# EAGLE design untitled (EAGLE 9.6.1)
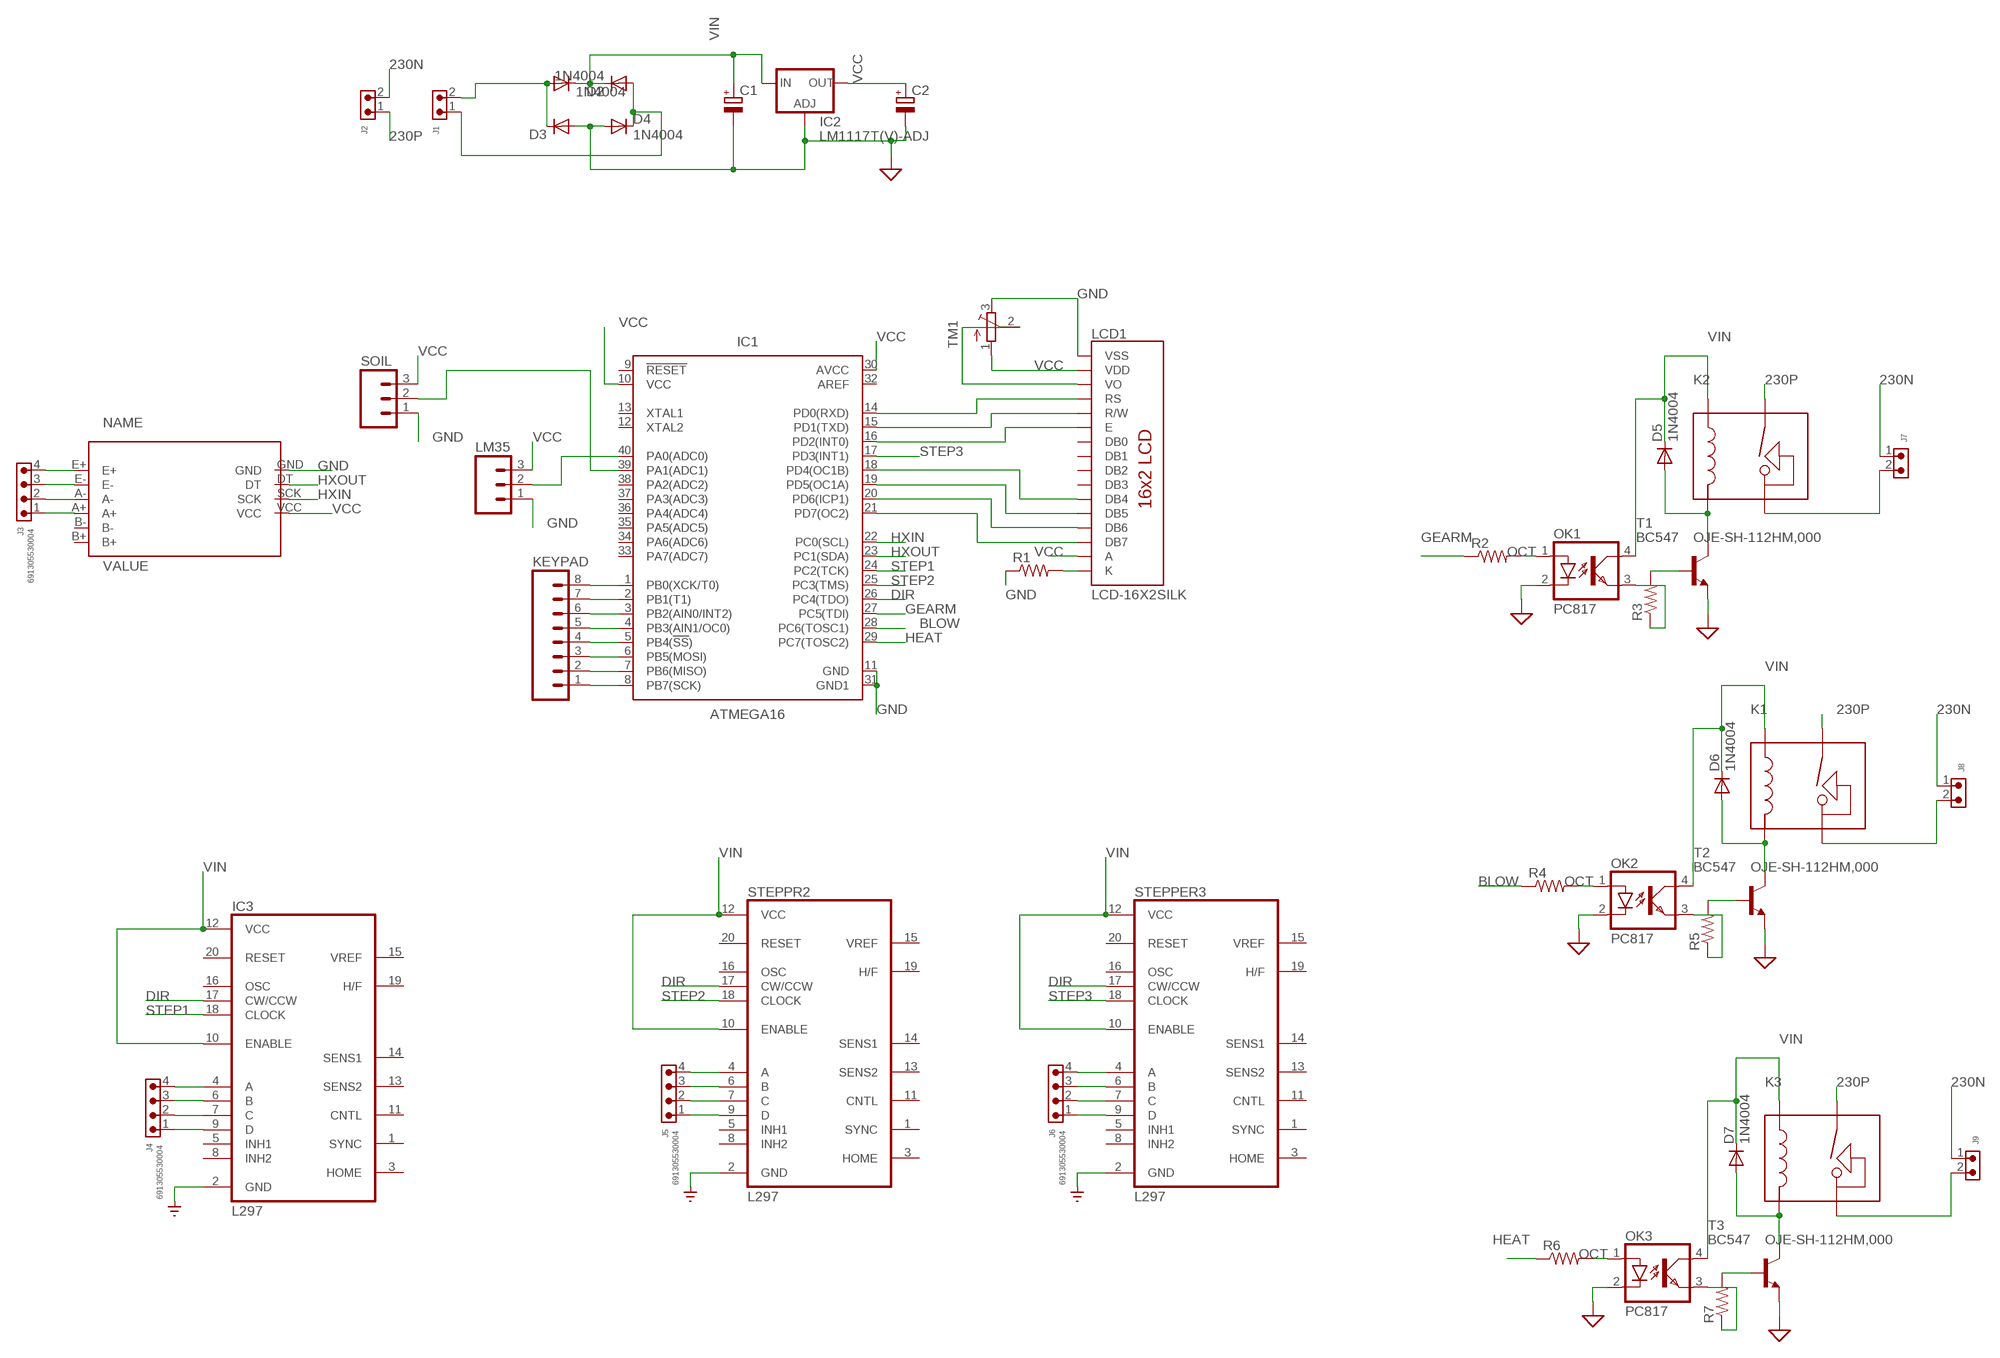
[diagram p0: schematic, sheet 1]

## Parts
C1  CPOL-EUE5-10.5  [E5-10,5]
C2  CPOL-EUE5-10.5  [E5-10,5]
D1  1N4004  [DO41-10]
D2  1N4004  [DO41-10]
D3  1N4004  [DO41-10]
D4  1N4004  [DO41-10]
D5  1N4004  [DO41-10]
D6  1N4004  [DO41-10]
D7  1N4004  [DO41-10]
IC1  ATMEGA16  ATMEGA32-16PU_DIP  [DIP1587W56P254L5229H482Q40B]
IC2  LM1117T(V)-ADJ  [TO220V]
IC3  L297  [DIL20]
J1  691305530002  [691305530002]
J2  691305530002  [691305530002]
J3  691305530004  691305530004  [691305530004]
J4  691305530004  691305530004  [691305530004]
J5  691305530004  691305530004  [691305530004]
J6  691305530004  691305530004  [691305530004]
J7  691305530002  [691305530002]
J8  691305530002  [691305530002]
J9  691305530002  [691305530002]
K1  OJE-SH-112HM,000  [OJE-SH-112HM,000]
K2  OJE-SH-112HM,000  [OJE-SH-112HM,000]
K3  OJE-SH-112HM,000  [OJE-SH-112HM,000]
KEYPAD  M08  [08P]
LCD1  LCD-16X2SILK  [LCD-16X2]
LM35  M03  [03P]
OK1  PC817  [DIL04]
OK2  PC817  [DIL04]
OK3  PC817  [DIL04]
R1  R-US_0207/9  [0207/9]
R2  R-US_0207/10  [0207/10]
R3  R-US_0207/10  [0207/10]
R4  R-US_0207/10  [0207/10]
R5  R-US_0207/10  [0207/10]
R6  R-US_0207/10  [0207/10]
R7  R-US_0207/10  [0207/10]
SOIL  M03  [03P]
STEPPER3  L297  [DIL20]
STEPPR2  L297  [DIL20]
T1  BC547  [TO92]
T2  BC547  [TO92]
T3  BC547  [TO92]
TM1  TRIMPOTTC33X  [TC33X]
U$3  HX711A  [HX711]

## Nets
230N: J2.2 J7.1 J8.1 J9.1
230P: J2.1 K1.NC K2.NC K3.NC
BLOW: IC1.28(PC6(TOSC1)) R4.1
DIR: IC1.26(PC4(TDO)) IC3.17(CW/CCW) STEPPER3.17(CW/CCW) STEPPR2.17(CW/CCW)
GEARM: IC1.27(PC5(TDI)) R2.1
GND: C1.- C2.- D3.A D4.A IC1.11(GND) IC1.31(GND1) IC2.1(ADJ) IC3.2(GND) LCD1.1(VSS) LM35.1 OK1.2(C) OK2.2(C) OK3.2(C) R1.1 SOIL.1 STEPPER3.2(GND) STEPPR2.2(GND) T1.1(E) T2.1(E) T3.1(E) TM1.3(E) U$3.GND ; supply symbol labelled SUP, SUPPLY0_GND_
HEAT: IC1.29(PC7(TOSC2)) R6.1
HXIN: IC1.22(PC0(SCL)) U$3.SCK
HXOUT: IC1.23(PC1(SDA)) U$3.DT
N$1: D1.A D3.C J1.2
N$2: D2.A D4.C J1.1
N$3: J3.4 U$3.E+
N$4: IC1.8(PB7(SCK)) KEYPAD.1
N$5: IC1.7(PB6(MISO)) KEYPAD.2
N$6: IC1.6(PB5(MOSI)) KEYPAD.3
N$7: IC1.5(PB4(!SS!)) KEYPAD.4
N$8: IC1.4(PB3(AIN1/OC0)) KEYPAD.5
N$9: J3.3 U$3.E-
N$10: J3.2 U$3.A-
N$11: J3.1 U$3.A+
N$12: IC1.3(PB2(AIN0/INT2)) KEYPAD.6
N$13: IC1.2(PB1(T1)) KEYPAD.7
N$14: IC1.1(PB0(XCK/T0)) KEYPAD.8
N$15: IC1.21(PD7(OC2)) LCD1.14(DB7)
N$16: IC1.20(PD6(ICP1)) LCD1.13(DB6)
N$17: IC1.19(PD5(OC1A)) LCD1.12(DB5)
N$18: IC1.18(PD4(OC1B)) LCD1.11(DB4)
N$19: IC1.14(PD0(RXD)) LCD1.4(RS)
N$20: IC1.15(PD1(TXD)) LCD1.5(R/W)
N$21: IC1.16(PD2(INT0)) LCD1.6(E)
N$22: IC3.4(A) J4.4
N$23: LCD1.3(VO) TM1.2(S)
N$24: IC3.6(B) J4.3
N$25: LCD1.16(K) R1.2
N$26: IC3.7(C) J4.2
N$27: IC3.9(D) J4.1
N$28: J5.4 STEPPR2.4(A)
N$29: J5.3 STEPPR2.6(B)
N$30: J5.2 STEPPR2.7(C)
N$31: J5.1 STEPPR2.9(D)
N$32: J6.4 STEPPER3.4(A)
N$33: J6.3 STEPPER3.6(B)
N$34: J6.2 STEPPER3.7(C)
N$35: J6.1 STEPPER3.9(D)
N$36: D5.A K2.A2 T1.3(C)
N$37: OK1.3(EMIT) R3.1
N$38: R3.2 T1.2(B)
N$39: IC1.40(PA0(ADC0)) LM35.2
N$40: J7.2 K2.NO
N$41: D6.A K1.A2 T2.3(C)
N$42: OK2.3(EMIT) R5.1
N$43: R5.2 T2.2(B)
N$44: IC1.39(PA1(ADC1)) SOIL.2
N$45: J8.2 K1.NO
N$46: D7.A K3.A2 T3.3(C)
N$47: OK3.3(EMIT) R7.1
N$48: R7.2 T3.2(B)
N$50: J9.2 K3.NO
OCT: OK1.1(A) OK2.1(A) OK3.1(A) R2.2 R4.2 R6.2
STEP1: IC1.24(PC2(TCK)) IC3.18(CLOCK)
STEP2: IC1.25(PC3(TMS)) STEPPR2.18(CLOCK)
STEP3: IC1.17(PD3(INT1)) STEPPER3.18(CLOCK)
VCC: C2.+ IC1.10(VCC) IC1.30(AVCC) IC2.2(OUT) LCD1.2(VDD) LCD1.15(A) LM35.3 SOIL.3 TM1.1(A) U$3.VCC
VIN: C1.+ D1.C D2.C D5.C D6.C D7.C IC2.3(IN) IC3.10(ENABLE) IC3.12(VCC) K1.A1 K2.A1 K3.A1 OK1.4(COL) OK2.4(COL) OK3.4(COL) STEPPER3.10(ENABLE) STEPPER3.12(VCC) STEPPR2.10(ENABLE) STEPPR2.12(VCC)
Unconnected: IC1.9(!RESET!) IC1.12(XTAL2) IC1.13(XTAL1) IC1.32(AREF) IC1.33(PA7(ADC7)) IC1.34(PA6(ADC6)) IC1.35(PA5(ADC5)) IC1.36(PA4(ADC4)) IC1.37(PA3(ADC3)) IC1.38(PA2(ADC2)) IC3.1(SYNC) IC3.3(HOME) IC3.5(INH1) IC3.8(INH2) IC3.11(CNTL) IC3.13(SENS2) IC3.14(SENS1) IC3.15(VREF) IC3.16(OSC) IC3.19(H/F) IC3.20(RESET) LCD1.7(DB0) LCD1.8(DB1) LCD1.9(DB2) LCD1.10(DB3) STEPPER3.1(SYNC) STEPPER3.3(HOME) STEPPER3.5(INH1) STEPPER3.8(INH2) STEPPER3.11(CNTL) STEPPER3.13(SENS2) STEPPER3.14(SENS1) STEPPER3.15(VREF) STEPPER3.16(OSC) STEPPER3.19(H/F) STEPPER3.20(RESET) STEPPR2.1(SYNC) STEPPR2.3(HOME) STEPPR2.5(INH1) STEPPR2.8(INH2) STEPPR2.11(CNTL) STEPPR2.13(SENS2) STEPPR2.14(SENS1) STEPPR2.15(VREF) STEPPR2.16(OSC) STEPPR2.19(H/F) STEPPR2.20(RESET) U$3.B+ U$3.B-

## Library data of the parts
C1 C2 = rcl:CPOL-EU: POLARIZED CAPACITOR, European symbol; SPICEPREFIX: C
D1-D7 = adafruit:1N4004: DIODE
IC1 = IC_Embedded:ATMEGA32*DIP: 8-bit Microcontroller with 32KBytes In-System Programmable Flash Datasheet; CATEGORY: IC_Embedded; DESCRIPTION: IC MCU 8BIT 32KB FLASH 40DIP; MANUFACTURER: Microchip Technology; MPN: ATMEGA32-16PU; OPERATING_TEMP: -40°C to 85°C; PART_STATUS: Active; SERIES: AVR® ATmega; SPEED: 16MHz; SUB-CATEGORY: Microcontroller
IC2 = lm1117_10:LM1117?-ADJ: 800mA Low-Dropout Linear Regulator Source: http://www.ti.com/lit/ds/symlink/lm1117-n.pdf; MF: Texas Instruments; MPN: LM1777T-ADJ; OC_FARNELL: 9485805; OC_NEWARK: 13B5345
IC3 STEPPER3 STEPPR2 = st-microelectronics:L297: STEPPER MOTOR CONTROLLER; MPN: L297/1; OC_FARNELL: 1094209; OC_NEWARK: 56P8258
J1 J2 J7-J9 = Wurth_Connectors_WR-TBL Pluggable Connector:691305530002: WR-TBL Serie 3055 - 5,08 mm - PCB Header Vertical Entry with Plastic Latches; DATASHEET-URL: https://www.we-online.com/catalog/datasheet/691305530002.pdf; IR-UL: 16A; MOUNT: THT; PART-NUMBER: 691305530002; PINS: 2; PITCH: 5.08mm; TYPE: Vertical; WORKING-VOLTAGE-UL: 300V (AC)
J3-J6 = Wurth_Connectors_WR-TBL Pluggable Connector:691305530004: WR-TBL Serie 3055 - 5,08 mm - PCB Header Vertical Entry with Plastic Latches KIND PROPERTIES Pitch 5.08 mm MATERIAL PROPERTIES Insulator Material PA66 Insulator Flammability Rating UL94 V-0 Insulator Color Green Terminal Material Copper Alloy Terminal Plating Tin-plated surface GENERAL INFORMATION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; DATASHEET-URL: https://www.we-online.com/catalog/datasheet/691305530004.pdf; IR-UL: 16A; MOUNT: THT; PART-NUMBER: 691305530004; PINS: 4; PITCH: 5.08mm; TYPE: Vertical; WORKING-VOLTAGE-UL: 300V (AC)
K1-K3 = Relay:OJE-SH-112HM,000: RELAY GEN PURPOSE SPST 10A 12V Manufacturer's datasheet; CREATED_BY: PCBLayout.com; DIGIKEY_PART_NUMBER: PB876-ND; MANUFACTURER: TE Connectivity Potter & Brumfield Relays; MANUFACTURER_PART_NUMBER: OJE-SH-112HM,000
KEYPAD = con-amp-quick:M08: AMP QUICK CONNECTOR; OC_FARNELL: unknown; OC_NEWARK: unknown
LCD1 = SparkFun-Displays:LCD-16X2: Standard text-only 16x2 parallel input LCD Basic 16 character by 2 line display. Typically utilizes the extremely common HD44780 parallel interface chipset SparkFun Products: Basic 16x2 Green Basic 8x2 Green; SF_ID: LCD-00255
LM35 SOIL = con-amp-quick:M03: AMP QUICK CONNECTOR; OC_FARNELL: unknown; OC_NEWARK: unknown
OK1-OK3 = optocoupler:PC817: SHARP OPTO COUPLER; MPN: PC817X4J000F; OC_FARNELL: 9707727; OC_NEWARK: 97K7059
R1-R7 = adafruit:R-US_: RESISTOR, American symbol
T1-T3 = transistor:BC547: NPN TRANSISTOR
TM1 = adafruit:TRIMPOT: SMT trimmer potentiometer part number TC33X http://www.ladyada.net/library/eagle
U$3 = HX711:HX711

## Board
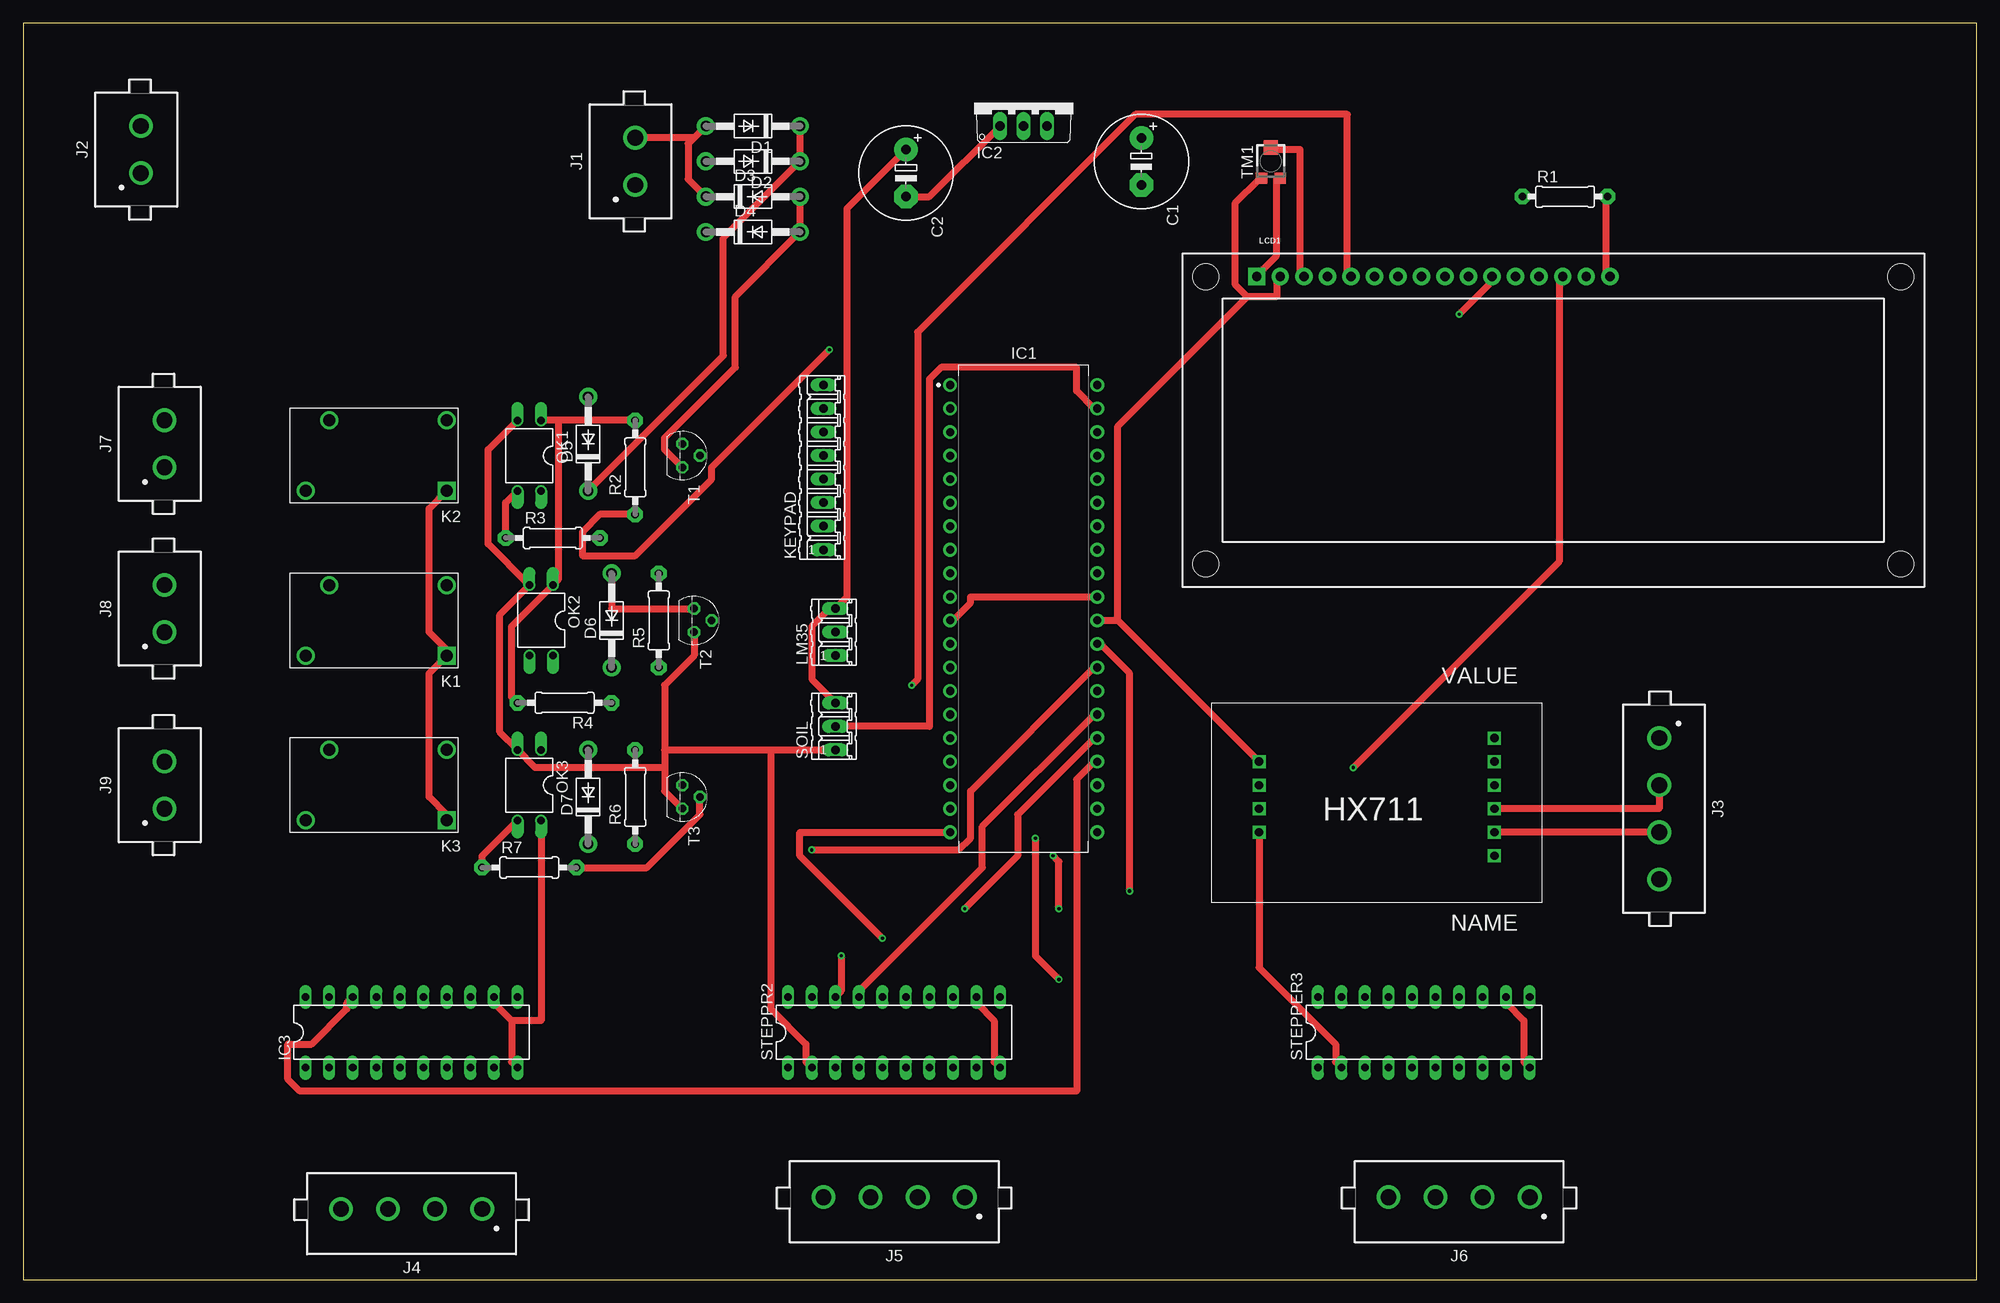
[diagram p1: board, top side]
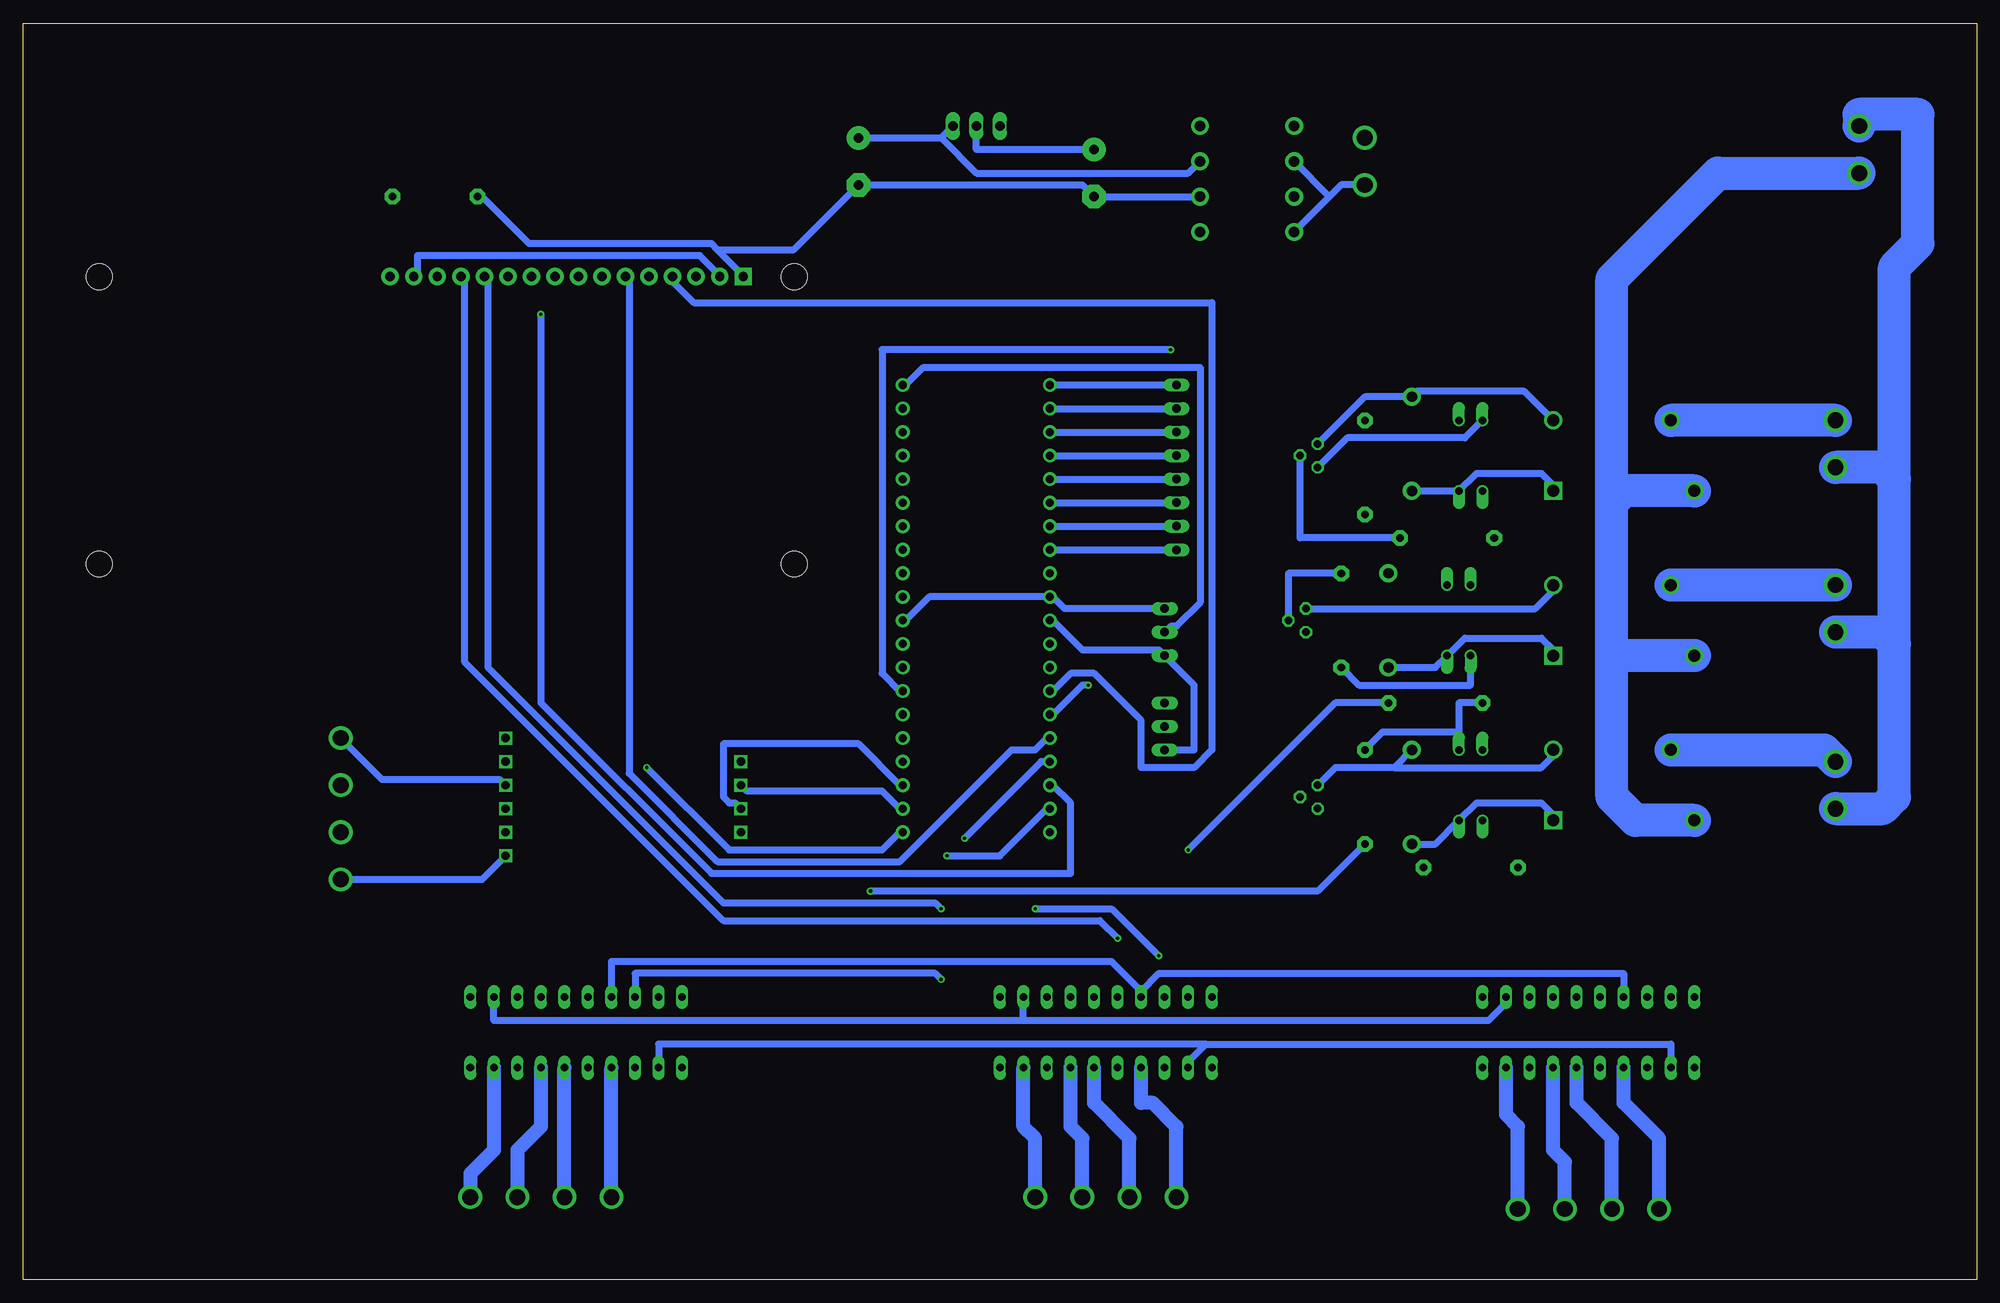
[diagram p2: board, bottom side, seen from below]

Size 210.8 x 135.56 mm. Coordinates in mm from the lower left corner, seen from the top.
Outline: 0,0 210.8,0 210.8,135.56 0,135.56 0,0
Copper layers (1*16): Top 0.035mm / dielectric 1.5mm / Bottom 0.035mm
Design rules "default *": minimum track width 30mil, minimum drill 0.35mm, track to track 20mil, track to pad 20mil, pad to pad 6mil, via to via 6mil, smd to smd 6mil, copper to edge 40mil, drill to drill 6mil, minimum pad ring 10mil, minimum via ring 8mil, stop-mask expansion 4mil, vias tented up to drill 0mil, thermal gap 10mil

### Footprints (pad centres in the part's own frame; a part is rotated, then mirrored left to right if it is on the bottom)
E5-10,5 = drill 1.016 pad 2.54: + -2.54,0 | drill 1.016 pad 2.54 octagon: - 2.54,0
DO41-10 = drill 1.118 pad 1.93: A 5.08,0; C -5.08,0
DIP1587W56P254L5229H482Q40B = drill 0.877 pad 1.477: 1 -7.938,24.13; 2 -7.938,21.59; 3 -7.938,19.05; 4 -7.938,16.51; 5 -7.938,13.97; 6 -7.938,11.43; 7 -7.938,8.89; 8 -7.938,6.35; 9 -7.938,3.81; 10 -7.938,1.27; 11 -7.938,-1.27; 12 -7.938,-3.81; 13 -7.938,-6.35; 14 -7.938,-8.89; 15 -7.938,-11.43; 16 -7.938,-13.97; 17 -7.938,-16.51; 18 -7.938,-19.05; 19 -7.938,-21.59; 20 -7.938,-24.13; 21 7.938,-24.13; 22 7.938,-21.59; 23 7.938,-19.05; 24 7.938,-16.51; 25 7.938,-13.97; 26 7.938,-11.43; 27 7.938,-8.89; 28 7.938,-6.35; 29 7.938,-3.81; 30 7.938,-1.27; 31 7.938,1.27; 32 7.938,3.81; 33 7.938,6.35; 34 7.938,8.89; 35 7.938,11.43; 36 7.938,13.97; 37 7.938,16.51; 38 7.938,19.05; 39 7.938,21.59; 40 7.938,24.13
TO220V = drill 1.016 long: 1 -2.54,-2.54; 2 0,-2.54; 3 2.54,-2.54
DIL20 = drill 0.813 long: 1 -11.43,-3.81; 2 -8.89,-3.81; 3 -6.35,-3.81; 4 -3.81,-3.81; 5 -1.27,-3.81; 6 1.27,-3.81; 7 3.81,-3.81; 8 6.35,-3.81; 9 8.89,-3.81; 10 11.43,-3.81; 11 11.43,3.81; 12 8.89,3.81; 13 6.35,3.81; 14 3.81,3.81; 15 1.27,3.81; 16 -1.27,3.81; 17 -3.81,3.81; 18 -6.35,3.81; 19 -8.89,3.81; 20 -11.43,3.81
691305530002 = drill 1.7: 1 -2.54,0; 2 2.54,0
691305530004 = drill 1.7: 1 -7.62,0; 2 -2.54,0; 3 2.54,0; 4 7.62,0
OJE-SH-112HM,000 = drill 1.3 square: A1 -7.62,3.8 | drill 1.3: A2 -7.62,-3.8; NC 7.62,3.8; NO 5.08,-3.8
08P = drill 0.914 long: 1 -8.89,0; 2 -6.35,0; 3 -3.81,0; 4 -1.27,0; 5 1.27,0; 6 3.81,0; 7 6.35,0; 8 8.89,0
LCD-16X2 = drill 1.016 pad 1.88 square: 1 -32,15.5 | drill 1.016 pad 1.88: 2 -29.46,15.5; 3 -26.92,15.5; 4 -24.38,15.5; 5 -21.84,15.5; 6 -19.3,15.5; 7 -16.76,15.5; 8 -14.22,15.5; 9 -11.68,15.5; 10 -9.14,15.5; 11 -6.6,15.5; 12 -4.06,15.5; 13 -1.52,15.5; 14 1.02,15.5; 15 3.56,15.5; 16 6.1,15.5 | hole 2.8: -37.5,15.5; -37.5,-15.5; 37.5,15.5; 37.5,-15.5
03P = drill 0.914 long: 1 -2.54,0; 2 0,0; 3 2.54,0
DIL04 = drill 0.813 offset: 1 -1.27,-3.81; 2 1.27,-3.81; 3 1.27,3.81; 4 -1.27,3.81
0207/9 = drill 0.813 pad 1.676 octagon: 1 -4.572,0; 2 4.572,0
0207/10 = drill 0.813 pad 1.676 octagon: 1 -5.08,0; 2 5.08,0
TO92 = drill 0.813 octagon: 1 1.27,0; 2 0,1.905; 3 -1.27,0
TC33X = smd 1.2 x 1.2: 1 -1,-1.825; 3 1,-1.825 | smd 1.5 x 1.6: 2 0,1.5
HX711 = drill 0.9 square: A+ 8.89,21.59; A- 8.89,24.13; B+ 8.89,16.51; B- 8.89,19.05; DT 34.29,24.13; E+ 8.89,29.21; E- 8.89,26.67; GND 34.29,26.67; SCK 34.29,21.59; VCC 34.29,19.05

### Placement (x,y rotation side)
C1  120.65,120.65 270 top
C2  95.25,119.38 270 top
D1  78.74,124.46 180 top
D2  78.74,120.65 180 top
D3  78.74,116.84 0 top
D4  78.74,113.03 0 top
D5  60.96,90.17 90 top
D6  63.5,71.12 90 top
D7  60.96,52.07 90 top
IC1  107.95,72.39 0 top
IC2  107.95,127 0 top
IC3  41.91,26.67 0 top
J1  66.04,120.65 90 top
J2  12.7,121.92 90 top
J3  176.53,50.8 270 top
J4  41.91,7.62 180 top
J5  93.98,8.89 180 top
J6  154.94,8.89 180 top
J7  15.24,90.17 90 top
J8  15.24,72.39 90 top
J9  15.24,53.34 90 top
K1  38.1,71.12 180 top
K2  38.1,88.9 180 top
K3  38.1,53.34 180 top
KEYPAD  86.36,87.63 90 top
LCD1  165.1,92.71 0 top
LM35  87.63,69.85 90 top
OK1  54.61,88.9 180 top
OK2  55.88,71.12 180 top
OK3  54.61,53.34 180 top
R1  166.37,116.84 0 top
R2  66.04,87.63 90 top
R3  57.15,80.01 0 top
R4  58.42,62.23 180 top
R5  68.58,71.12 90 top
R6  66.04,52.07 90 top
R7  54.61,44.45 0 top
SOIL  87.63,59.69 90 top
STEPPER3  151.13,26.67 0 top
STEPPR2  93.98,26.67 0 top
T1  71.12,88.9 270 top
T2  72.39,71.12 270 top
T3  71.12,52.07 270 top
TM1  134.62,120.65 0 top
U$3  167.64,74.93 180 top

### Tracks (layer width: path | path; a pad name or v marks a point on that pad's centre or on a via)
230N
  Bottom 3.556: J9.1 10.16,50.8 8.89,52.07 8.89,68.58 | 8.89,68.58 10.16,69.85 J8.1 | 8.89,68.58 8.89,86.36 | 8.89,86.36 10.16,87.63 J7.1 | 8.89,86.36 8.89,109.22 6.35,111.76 6.35,125.73 12.7,125.73 J2.2
230P
  Bottom 0.762: 38.1,67.31 39.37,67.31
  Bottom 3.556: K3.NC 36.83,49.53 39.37,52.07 39.37,67.31 39.37,83.82 | 39.37,83.82 39.37,107.95 27.94,119.38 J2.1 | K2.NC 38.1,85.09 39.37,83.82 | K1.NC 38.1,67.31
BLOW  (via drill 0.35)
  Top 0.762: v85.09,46.35 100.97,46.35 102.24,47.62 102.24,52.7 115.57,66.04 IC1.28
  Bottom 0.762: v85.09,46.35 69.22,62.23 R4.1
DIR
  Top 0.762: STEPPR2.17 90.17,31.11 103.5,44.45 103.5,48.9 115.57,60.96 IC1.26
  Bottom 0.762: IC3.17 38.1,33.02 88.26,33.02 90.17,31.11 | STEPPER3.17 147.32,34.29 93.34,34.29 90.17,31.11 | 90.17,31.11 STEPPR2.17
GEARM  (via drill 0.35)
  Top 0.762: v87,100.33 74.3,87.63 74.3,86.36 66.04,78.11 60.33,78.11 60.33,80.64 62.23,82.55 R2.1
  Bottom 0.762: v87,100.33 118.11,100.33 118.11,65.41 116.21,63.5 IC1.27
GND
  Top 0.762: STEPPER3.2 141.61,23.5 141.61,25.4 133.35,33.66 U$3.GND | D3.A D4.A 76.84,106.05 76.84,98.42 69.22,90.81 69.22,89.53 T1.1 | IC2.1 97.79,116.84 C2.- | TM1.3 135.25,118.75 135.25,110.49 133.35,108.58 LCD1.1 | IC1.31 102.24,73.66 102.24,73.03 100.33,71.12 IC1.11 | T3.1 69.22,52.7 69.22,55.24 | 69.22,57.15 69.22,64.14 72.39,67.31 T2.1 | 69.22,57.15 69.22,55.24 | 69.22,55.24 55.24,55.24 OK3.2 51.44,59.05 51.44,71.75 OK2.2 50.16,79.38 50.16,89.53 OK1.2 | 69.22,57.15 80.65,57.15 | 80.65,57.15 SOIL.1 | STEPPR2.2 84.46,23.5 84.46,25.4 80.65,29.21 80.65,57.15
  Bottom 0.762: IC3.2 33.02,25.4 83.19,25.4 | 83.19,25.4 85.09,23.5 STEPPR2.2 | STEPPER3.2 142.24,25.4 83.19,25.4 | D3.A C2.- 96.52,118.11 C1.- 127.63,111.12 135.89,111.12 | 135.89,111.12 133.35,108.58 LCD1.1 | 135.89,111.12 136.53,111.76 156.21,111.76 161.29,116.84 R1.1 | IC1.11 99.69,71.12 96.52,67.94 88.26,67.94 LM35.1 84.46,64.14 84.46,57.15 SOIL.1 | T1.1 67.94,90.81 55.24,90.81 OK1.2
HEAT  (via drill 0.35)
  Top 0.762: v119.38,41.91 119.38,65.41 116.21,68.58 IC1.29
  Bottom 0.762: v119.38,41.91 71.12,41.91 R6.1
HXIN
  Bottom 0.762: U$3.SCK 132.72,52.7 118.11,52.7 116.21,50.8 IC1.22
HXOUT
  Bottom 0.762: U$3.DT 133.99,51.44 134.62,51.44 135.25,52.07 135.25,57.78 120.65,57.78 116.21,53.34 IC1.23
N$1
  Top 0.762: D3.C 71.75,118.75 71.75,122.56 72.39,123.19 | D1.A 72.39,123.19 | 72.39,123.19 J1.2
N$2
  Bottom 0.762: 69.85,116.84 68.58,118.11 J1.1 | 69.85,116.84 D4.C | 69.85,116.84 D2.A
N$3
  Bottom 0.762: U$3.E+ 161.29,43.18 J3.4
N$4
  Bottom 0.762: IC1.8 KEYPAD.1
N$5
  Bottom 0.762: IC1.7 KEYPAD.2
N$6
  Bottom 0.762: IC1.6 KEYPAD.3
N$7
  Bottom 0.762: IC1.5 KEYPAD.4
N$8
  Bottom 0.762: IC1.4 KEYPAD.5
N$9
  Top 0.762: J3.3 U$3.E-
N$10
  Top 0.762: U$3.A- 176.53,50.8 J3.2
N$11
  Bottom 0.762: U$3.A+ 159.39,53.98 172.09,53.98 J3.1
N$12
  Bottom 0.762: IC1.3 KEYPAD.6
N$13
  Bottom 0.762: IC1.2 KEYPAD.7
N$14
  Bottom 0.762: IC1.1 KEYPAD.8
N$15  (via drill 0.35)
  Top 0.762: v143.51,55.24 165.74,77.47 165.74,107.95 LCD1.14
  Bottom 0.762: v143.51,55.24 134.62,46.35 118.11,46.35 116.21,48.26 IC1.21
N$16  (via drill 0.35)
  Top 0.762: IC1.20 83.82,48.26 83.82,45.72 v92.71,36.83
  Bottom 0.762: v92.71,36.83 94.62,38.73 135.25,38.73 163.19,66.67 163.19,107.95 LCD1.13
N$17  (via drill 0.35)
  Top 0.762: v111.12,45.72 111.76,45.09 v111.76,40.01
  Bottom 0.762: v111.12,45.72 105.41,45.72 100.33,50.8 IC1.19 | v111.76,40.01 112.4,40.64 135.25,40.64 160.66,66.04 160.66,107.95 LCD1.12
N$18  (via drill 0.35)
  Top 0.762: v154.94,104.14 158.12,107.31 158.12,107.95 LCD1.11
  Bottom 0.762: v154.94,104.14 154.94,62.23 136.53,43.81 97.79,43.81 97.79,51.44 99.69,53.34 IC1.18
N$19
  Bottom 0.762: IC1.14 99.69,63.5 97.79,65.41 95.25,65.41 90.17,60.33 90.17,55.24 84.46,55.24 82.55,57.15 82.55,105.41 138.43,105.41 140.97,107.95 LCD1.4
N$20  (via drill 0.35)
  Top 0.762: v95.88,64.14 96.52,64.77 96.52,102.23 120.01,125.73 142.88,125.73 142.88,108.58 LCD1.5
  Bottom 0.762: v95.88,64.14 96.52,64.14 99.69,60.96 IC1.15
N$21
  Bottom 0.762: IC1.16 100.33,58.42 101.6,57.15 104.14,57.15 116.21,45.09 135.89,45.09 145.42,54.61 145.42,107.95 LCD1.6
N$22
  Bottom 1.524: J4.4 34.29,15.24 38.1,19.05 IC3.4
N$23
  Top 0.762: TM1.2 134.62,121.92 137.79,121.92 137.79,108.58 LCD1.3
N$24
  Bottom 1.524: IC3.6 43.18,19.05 39.37,15.24 J4.3
N$25
  Top 0.762: R1.2 170.81,116.84 170.81,108.58 LCD1.16
N$26
  Bottom 1.524: J4.2 44.45,12.7 45.72,13.97 IC3.7
N$27
  Bottom 1.524: J4.1 49.53,16.51 50.8,17.78 IC3.9
N$28
  Bottom 1.524: J5.4 86.36,16.51 88.9,19.05 90.17,19.05 STEPPR2.4
N$29
  Bottom 1.524: STEPPR2.6 95.25,19.05 91.44,15.24 J5.3
N$30
  Bottom 1.524: STEPPR2.7 97.79,16.51 96.52,15.24 J5.2
N$31
  Bottom 1.524: J5.1 101.6,15.24 102.87,16.51 STEPPR2.9
N$32
  Bottom 1.524: J6.4 STEPPER3.4
N$33
  Bottom 1.524: J6.3 STEPPER3.6
N$34
  Bottom 1.524: J6.2 157.48,13.97 154.94,16.51 STEPPER3.7
N$35
  Bottom 1.524: J6.1 162.56,11.43 160.02,13.97 STEPPER3.9
N$36
  Bottom 0.762: T1.3 66.04,95.25 D5.A 60.33,95.89 48.9,95.89 K2.A2
N$37
  Top 0.762: OK1.3 52.07,83.82 R3.1
N$38
  Bottom 0.762: T1.2 73.03,80.01 R3.2
N$39
  Bottom 0.762: LM35.2 87,70.48 86.36,70.48 83.82,73.03 83.82,98.42 113.66,98.42 115.57,96.52 IC1.40
N$40
  Bottom 3.556: J7.2 K2.NO
N$41
  Top 0.762: T2.3 63.5,72.39 D6.A
  Bottom 0.762: T2.3 47.62,72.39 45.72,74.3 K1.A2
N$42
  Bottom 0.762: OK2.3 54.61,64.14 66.67,64.14 R5.1
N$43
  Bottom 0.762: T2.2 74.3,76.2 R5.2
N$44
  Top 0.762: SOIL.2 97.79,59.69 97.79,97.16 99.06,98.42 113.66,98.42 113.66,95.89 115.57,93.98 IC1.39
N$45
  Bottom 3.556: J8.2 K1.NO
N$46
  Bottom 0.762: T3.3 69.22,55.24 62.87,55.24 | D7.A 62.87,55.24 | 62.87,55.24 46.99,55.24 45.72,56.52 K3.A2
N$47
  Top 0.762: OK3.3 49.53,45.72 R7.1
N$48
  Top 0.762: T3.2 73.03,50.16 67.31,44.45 R7.2
N$50
  Bottom 3.556: K3.NO 16.5,57.14 J9.2
OCT
  Top 0.762: R2.2 57.78,92.71 | 57.78,92.71 OK1.1 | R4.2 52.7,62.87 52.7,70.48 OK2.1 57.78,75.56 57.78,92.71
  Bottom 0.762: 55.88,59.05 55.88,62.23 R4.2 | R6.2 64.13,59.05 55.88,59.05 | 55.88,59.05 OK3.1
STEP1
  Top 0.762: IC3.18 34.92,29.84 34.92,29.21 31.11,25.4 28.57,25.4 28.57,21.59 29.84,20.32 113.66,20.32 113.66,53.98 115.57,55.88 IC1.24
STEP2  (via drill 0.35)
  Top 0.762: STEPPR2.18 88.26,31.11 v88.26,34.92 | v101.6,40.01 107.31,45.72 107.31,50.16 115.57,58.42 IC1.25
  Bottom 0.762: v88.26,34.92 93.34,40.01 v101.6,40.01
STEP3  (via drill 0.35)
  Top 0.762: v111.76,32.38 109.22,34.92 v109.22,47.62
  Bottom 0.762: STEPPER3.18 144.78,33.02 112.4,33.02 v111.76,32.38 | v109.22,47.62 100.97,55.88 IC1.17
VCC
  Top 0.762: 132.08,106.05 130.81,107.31 130.81,116.2 133.35,118.75 TM1.1 | 132.08,106.05 135.25,106.05 135.25,107.95 LCD1.2 | 118.11,71.12 U$3.VCC | IC1.30 118.11,71.12 | SOIL.3 85.09,64.77 85.09,70.48 87,72.39 LM35.3 88.9,73.66 88.9,115.57 C2.+ | 132.08,106.05 118.11,92.08 118.11,71.12
  Bottom 0.762: LCD1.15 168.28,108.58 168.28,110.49 137.79,110.49 135.89,108.58 LCD1.2 | IC2.2 107.95,121.92 C2.+ | LM35.3 98.43,72.39 99.69,73.66 IC1.10 113.03,73.66 115.57,71.12 IC1.30
VIN
  Top 0.762: D1.C D2.C 75.56,112.39 75.56,99.69 D5.C | K2.A1 43.81,83.19 43.81,69.85 45.72,67.94 K1.A1 43.81,65.41 43.81,52.07 45.72,50.16 K3.A1 | STEPPER3.10 161.93,23.5 161.93,27.94 160.02,29.84 STEPPER3.12 | STEPPR2.10 104.78,23.5 104.78,27.94 102.87,29.84 STEPPR2.12 | IC3.10 52.7,23.5 52.7,27.94 | 52.7,27.94 50.8,29.84 IC3.12 | 52.7,27.94 55.88,27.94 OK3.4
  Bottom 0.762: 111.76,123.19 IC2.3 | C1.+ 111.76,123.19 | D2.C 85.09,119.38 107.95,119.38 111.76,123.19 | D5.C OK1.4 53.98,87 46.99,87 45.72,85.72 K2.A1 | D6.C 58.42,66.04 OK2.4 55.24,69.22 46.99,69.22 45.72,67.94 K1.A1 | D7.C 58.42,46.99 OK3.4 53.98,51.44 46.99,51.44 45.72,50.16 K3.A1 | 102.87,27.94 STEPPR2.12 | 102.87,27.94 52.7,27.94 50.8,29.84 IC3.12 | STEPPER3.12 160.02,27.94 102.87,27.94

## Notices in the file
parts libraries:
Wurth_Connectors_WR-TBL Pluggable Connec: Copyright: Würth Elektronik
SparkFun-Displays: Licensing: Creative Commons ShareAlike 4.0 International - https://creativecommons.org/licenses/by-sa/4.0
